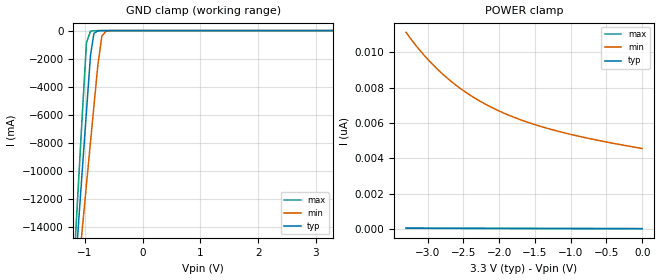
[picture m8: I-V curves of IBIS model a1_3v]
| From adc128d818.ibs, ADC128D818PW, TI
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[Model] a1_3v
Model_type Input
Vinh = 2.0V
Vinl = 0.8V
C_comp   1.18pF   1.09pF   1.34pF
[Voltage Range]   3.3V   3.0V   3.6V
[Temperature Range]   25.0   125.0   -40.0
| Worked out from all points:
|   GND clamp passes 1 mA (typ) near -0.65 V on its own axis
[GND Clamp]
-3.3V     -140.9A    -112.5A    -173A
-1.171V   -17.28A    -19.67A    -15.31A
-1.102V   -13.23A    -16.62A    -10.16A
-1.043V   -9.774A    -14.01A    -5.763A
-973.5mV  -5.764A    -10.98A    -872.2mA
-904.2mV  -1.783A    -7.965A    -42.01mA
-844.8mV  -197.3mA   -5.398A    -8.068mA
-775.5mV  -19.36mA   -2.42A     -2.167mA
-706.2mV  -3.206mA   -385.4mA   -450.9uA
-636.9mV  -646.1uA   -55.93mA   -65.71uA
-438.9mV  -3.11uA    -355uA     -57.03nA
3.293V    21.88pA    0A         19.76pA
[POWER Clamp]
-3.3V     49.64pA    11.13nA    41.58pA
-3.161V   47.87pA    10.38nA    40.75pA
-3.033V   46.33pA    9.768nA    39.98pA
-2.765V   43.37pA    8.687nA    38.37pA
-2.627V   41.96pA    8.219nA    37.54pA
-2.458V   40.33pA    7.722nA    36.53pA
-2.3V     38.88pA    7.316nA    35.58pA
-2.092V   37.07pA    6.86nA     34.33pA
-1.696V   33.87pA    6.18nA     31.96pA
-1.261V   30.62pA    5.627nA    29.34pA
-696.3mV  26.64pA    5.087nA    25.96pA
-3.3mV    21.95pA    4.562nA    21.8pA
